FUNCTION_BLOCK FB99
TITLE =Set Operation Mode
//*****************************************************************************
//* maxon motor ag
//* R&D
//* all rights reserved
//*****************************************************************************
//* Summary:  SetOperation Mode
//*
//* Remarks:
//*
//* Created under: STEP7 REV5.2+SP1
//*****************************************************************************
//* History:
//* 18.05.2004 | INA   first release
//*
//*
//*****************************************************************************
//

AUTHOR:INA
FAMILY:StateMac
NAME:SetOpMod
VERSION:00.01


VAR_INPUT

Write : BOOL //A rising edge start the command

  NodeID : BYTE //Adress of the maxon device

  Mode : BYTE //Operation Mode

END_VAR
VAR_OUTPUT
  Done : BOOL //Data valid flag is TRUE if data were available

  Err : BOOL //Error flag is TRUE if an Error has occured, see ErrNo for more details

  ErrNo : DINT //Contains detailed error information

END_VAR
VAR
  xEdgeMerker : BOOL //Edge Merker

  xEdgeFlag : BOOL //Edge Flag

  xStep : INT
END_VAR

BEGIN

NETWORK
TITLE = Activate the service function
//

// SDO Write "Set Operation Mode"

       U    #Write
       FP   #xEdgeFlag                   // recognize a positiv edge of the Read signal
       =    #xEdgeMerker                 // and set the xEdgeMerker for one cycle to true

       L    #xStep
       L    0
       ==I
       U    #xEdgeMerker
       SPB  nstp                         // iStep = 1 -> fnc1

       L    #xStep                       // jump list
       SPL  List
       SPA  rdef
       SPA  fnc1
       SPA  fncE
List  :SPA  rdef

rdef  :NOP  0
       R    #Done                        // reset Done
       R    #Err
       L    0
       T    #xStep                       // iStep = 0
       SPA  end

fnc1  :NOP  0

       CALL FC14
         NodeID:=#NodeID
         Index:=DW#16#00006060
         SubIndex:=DW#16#00000000
         ValueIn:=#Mode
         RET_VAL:=#Done
         Err:=#Err
         ErrNo:=#ErrNo

fncE  :NOP  0
       L    0
       T    #xStep
       SPA  end

nstp  :NOP  0
       L    #xStep
       INC            1
       T    #xStep

end   :NOP  0
END_FUNCTION_BLOCK
